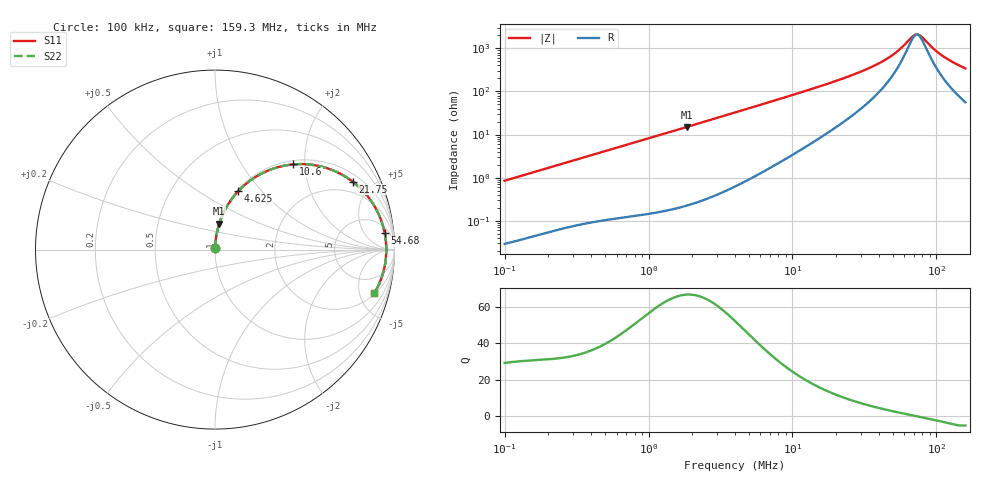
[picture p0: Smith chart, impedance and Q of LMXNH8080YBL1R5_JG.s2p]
! LMXNH8080YBL1R5_JG  S-PARAMETER MODEL  ( Standard Model )
! Model Generated by TAIYO YUDEN Corporation (http://www.ty-top.com)
! Version 1.0
! TAIYO YUDEN Control No. 20240226
! Copyright(c) 2024 TAIYO YUDEN CO.,LTD. All Rights Reserved.
! Product Description (link to TY-COMPAS)
! https://ds.yuden.co.jp/TYCOMPAS/or/detail?pn=LMXNH8080YBL1R5NJG&u=M
! Products Name : Inductors
! Characteristics :
!  Inductance : 1.5 [uH] , SRF(min) : 63 [MHz] , DC Resistance(max) : 0.0091 [Ohm]
!  Rated Current : Saturation  10000 [mA] , Temp Rise  7000 [mA] (40 [degC])
!  Case Size : 8.0 x 8.0 / 0.315 x 0.315 [mm/inch] , Thickness : 4.2 / 0.165 [mm/inch]
!  (Conditions: Temperature = 25 [degC] , DC Bias Current = 0 [A])
! External Node Assignments :
!  1  o---GGG---o  2
! GND o---------o GND
! Frequency Range : 0.1MHz  -  159.254811MHz  [ 402 STEP ]
# MHz S RI R 50
! Freq[MHz].  S11 Real  S11 Imag  S21 Real  S21 Imag  S12 Real  S12 Imag  S22 Real  S22 Imag
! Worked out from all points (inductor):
!   401 points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, 100 kHz to 159.3 MHz, reference 50 ohm
!   read as one part in series: L = 1.34 uH near 103.8 kHz
!   highest Q = 66.7 at 1.84 MHz (marker M1), where L = 1.29 uH
!   self-resonance near 73.36 MHz
!   S11 on the Smith chart (normalised r, x): 100 kHz: 1.00, +0.02; 4.625 MHz: 1.02, +0.75; 10.6 MHz: 1.08, +1.75; 21.75 MHz: 1.36, +3.83; 54.68 MHz: 9, +16; 159.3 MHz: 2.12, -6.77
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0.1  0.000361 0.00846  0.9996 -0.00846  0.9996 -0.00846  0.000361 0.00846
0.343835  0.00163 0.0283  0.9984 -0.0283  0.9984 -0.0283  0.00163 0.0283
1.182227  0.0107 0.0949  0.9893 -0.0949  0.9893 -0.0949  0.0107 0.0949
1.840037  0.0239 0.1454  0.9761 -0.1454  0.9761 -0.1454  0.0239 0.1454
2.863862  0.0544 0.2189  0.9456 -0.2189  0.9456 -0.2189  0.0544 0.2189
4.064915  0.103 0.2944  0.897 -0.2944  0.897 -0.2944  0.103 0.2944
4.624749  0.1291 0.3249  0.8709 -0.3249  0.8709 -0.3249  0.1291 0.3249
6.937504  0.2495 0.4184  0.7505 -0.4184  0.7505 -0.4184  0.2495 0.4184
10.60043  0.4371 0.4749  0.5629 -0.4749  0.5629 -0.4749  0.4371 0.4749
13.72135  0.5659 0.4684  0.4341 -0.4684  0.4341 -0.4684  0.5659 0.4684
21.75342  0.7671 0.3788  0.2329 -0.3788  0.2329 -0.3788  0.7671 0.3788
33.85736  0.8878 0.2431  0.1122 -0.2431  0.1122 -0.2431  0.8878 0.2431
47.17884  0.9344 0.1368  0.0656 -0.1368  0.0656 -0.1368  0.9344 0.1368
54.67504  0.9458 0.0906  0.0542 -0.0906  0.0542 -0.0906  0.9458 0.0906
68.21061  0.954 0.0223  0.046 -0.0223  0.046 -0.0223  0.954 0.0223
72.08877  0.9545 0.00537  0.0455 -0.00537  0.0455 -0.00537  0.9545 0.00537
74.79595  0.9545 -0.00593  0.0455 0.00593  0.0455 0.00593  0.9545 -0.00593
79.04852  0.954 -0.0229  0.046 0.0229  0.046 0.0229  0.954 -0.0229
95.04868  0.9478 -0.0797  0.0522 0.0797  0.0522 0.0797  0.9478 -0.0797
110.1509  0.9377 -0.1258  0.0623 0.1258  0.0623 0.1258  0.9377 -0.1258
132.4464  0.9175 -0.1844  0.0825 0.1844  0.0825 0.1844  0.9175 -0.1844
159.2548  0.8876 -0.2438  0.1124 0.2438  0.1124 0.2438  0.8876 -0.2438
